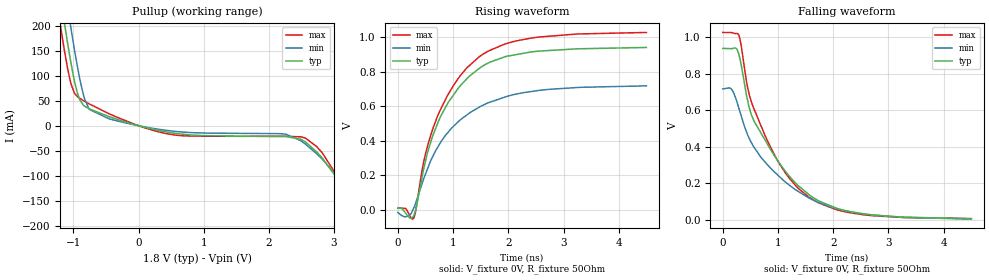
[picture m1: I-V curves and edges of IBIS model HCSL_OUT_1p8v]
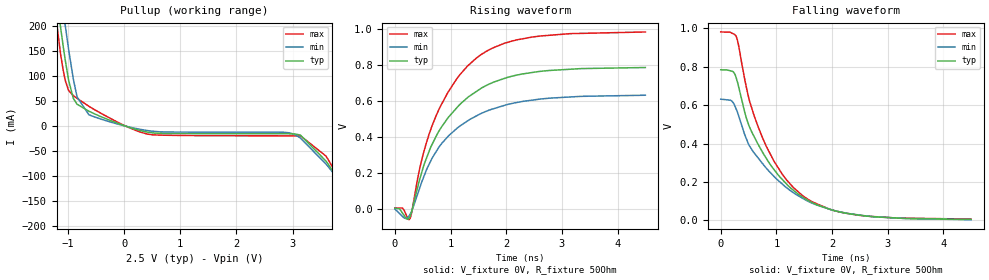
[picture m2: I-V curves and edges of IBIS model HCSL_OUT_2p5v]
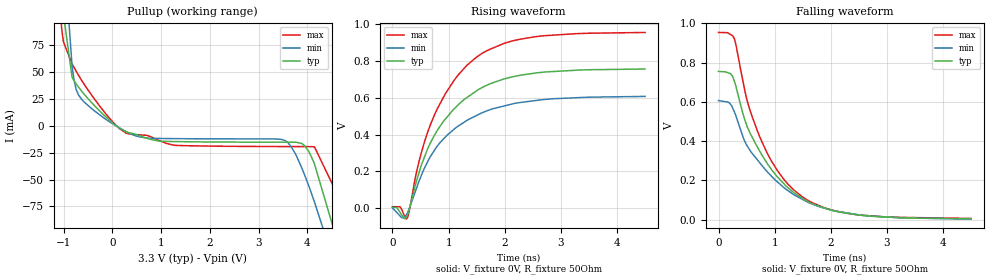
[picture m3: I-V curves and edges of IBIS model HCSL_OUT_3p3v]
|Texas Instruments Incorporated
|Storage Products Group
| Marketing part#   Voltage Range   Package-type   #pins
| CDCUN1208LP   1.7 to  3.63V   QFN   32
[IBIS Ver]   4.0
[File name]   cdcun1208lp.ibs
[File Rev]   1.1
[Date]   04/12/2012
[Source]   Texas Instruments Incorporated.
|   Analog-eLab, HPA
|   12500 TI Blvd
|   Dallas, TX -75243
|   For Support e-mail: elab_ibis@list.ti.com
[Notes]
|-Revision History:
| 1.0: 4/12/2012
| - Initial version of the model
| - Initial Model generated from simulations in TISPICE
| - No syntax warnings or errors based on the
| committee parser checker
| For UNIV_IN2 model, the internal on-chip 50 ohm termination to ground (for
| a HCSL input) and 50 ohm termination to 1.2V (for
| a LVDS input) are not represented in this file. It is recommended
| that a user,who wished to see the benefit of these on-chip terminations,
| implement an appropriate termination explicitly on the final simulation
| level as needed.
[Disclaimer]
 This product is designed as an aid for customers of Texas Instruments.
 No warranties, either expressed or implied, with respect to this third
 party software (if any) or with respect to its fitness for any
 particular purpose is claimed by Texas Instruments or the author. The
 software (if any) is provided solely on an "as is" basis. The entire
 risk as to its quality and performance is with the customer
[Copyright] (C) Copyright 2012 Texas Instruments Incorporated.
   All rights reserved.
|   Component  CDCUN1208LP
[Component]   CDCUN1208LP
[Manufacturer]   Texas Instruments Incorporated
[Package]
| 32-pin QFN
|   typ   min   max
R_pkg   0.44   0.40   0.47
L_pkg   0.734nH   0.634nH   0.824nH
C_pkg   185fF   175fF   195fF
[Pin]   signal_name   model_name   R_pin   L_pin   C_pin
1   DIVIDE   NC   NA   NA   NA
2   INSEL   NC   NA   NA   NA
3   IN1P   UNIV_IN2   NA   NA   NA
4   IN1N   UNIV_IN2   NA   NA   NA
5   VDD   POWER   NA   NA   NA
6   IN2P   UNIV_IN2   NA   NA   NA
7   IN2N   UNIV_IN2   NA   NA   NA
8   ITTP   NC   NA   NA   NA
9   OUT1P   UNIV_OUT   NA   NA   NA
10   OUTIN   UNIV_OUT   NA   NA   NA
11   VDDO1   POWER   NA   NA   NA
12   OUT2P   UNIV_OUT   NA   NA   NA
13   OUT2N   UNIV_OUT   NA   NA   NA
14   VDDO2   POWER   NA   NA   NA
15   OUT3P   UNIV_OUT   NA   NA   NA
16   OUT3N   UNIV_OUT   NA   NA   NA
17   OUT4P   UNIV_OUT   NA   NA   NA
18   OUT4N   UNIV_OUT   NA   NA   NA
19   OTTP   NC   NA   NA   NA
20   OUT5P   UNIV_OUT   NA   NA   NA
21   OUT5N   UNIV_OUT   NA   NA   NA
22   VDDO3   POWER   NA   NA   NA
23   OUT6P   UNIV_OUT   NA   NA   NA
24   OUT6N   UNIV_OUT   NA   NA   NA
25   OUT7P   UNIV_OUT   NA   NA   NA
26   OUT7N   UNIV_OUT   NA   NA   NA
27   VDDO4   POWER   NA   NA   NA
28   OUT8P   UNIV_OUT   NA   NA   NA
29   OUT8N   UNIV_OUT   NA   NA   NA
30   MODE   NC   NA   NA   NA
31   ERC   NC   NA   NA   NA
32   OE   NC   NA   NA   NA
[Diff Pin]  inv_pin  vdiff  tdelay_typ tdelay_min tdelay_max
3   4   200mV   NA   NA   NA
6   7   200mV   NA   NA   NA
9   10   NA   NA   NA   NA
12   13   NA   NA   NA   NA
15   16   NA   NA   NA   NA
17   18   NA   NA   NA   NA
20   21   NA   NA   NA   NA
23   24   NA   NA   NA   NA
25   26   NA   NA   NA   NA
28   29   NA   NA   NA   NA
[Model Selector]   UNIV_OUT
HCSL_OUT_1p8v   HCSL driver w/ 1.8V supply
HCSL_OUT_2p5v   HCSL driver w/ 2.5V supply
HCSL_OUT_3p3v   HCSL driver w/ 3.3V supply
LVCMOS_OUT_1p8v   LVCMOS driver w/ 1.8V supply
LVCMOS_OUT_2p5v   LVCMOS driver w/ 2.5V supply
LVCMOS_OUT_3p3v   LVCMOS driver w/ 3.3V supply
LVDS_OUT_1p8v   LVDS driver w/ 1.8V supply
LVDS_OUT_2p5v   LVDS driver w/ 2.5V supply
LVDS_OUT_3p3v   LVDS driver w/ 3.3V supply
[Model Selector]   IN1
IN1_1p8v   input1 w/ 1.8V supply
IN1_2p5v   input1 w/ 2.5V supply
IN1_3p3v   input1 w/ 3.3V supply
[Model Selector]   UNIV_IN2
UNIVIN2_1p8v   Universal input w/ 1.8V supply
UNIVIN2_2p5v   Universal input w/ 2.5V supply
UNIVIN2_3p3v   Universal input w/ 3.3V supply
| Models and submodels in the file (15): HCSL_OUT_1p8v (Open_source), HCSL_OUT_2p5v (Open_source), HCSL_OUT_3p3v (Open_source), LVCMOS_OUT_1p8v (Output), LVCMOS_OUT_2p5v (Output), LVCMOS_OUT_3p3v (Output), LVDS_OUT_1p8v (Output), LVDS_OUT_2p5v (Output), LVDS_OUT_3p3v (Output), IN1_1p8v (Input), IN1_2p5v (Input), IN1_3p3v (Input), UNIVIN2_1p8v (Input), UNIVIN2_2p5v (Input), UNIVIN2_3p3v (Input)
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[Model]   HCSL_OUT_1p8v
Model_type   Open_source
Polarity   Non-Inverting
Vmeas = 0.35
Vref = 0
Cref = 0pF
Rref = 50
|   typ   min   max
C_comp   1pF   1pF   1pF
[Voltage Range]   1.8   1.7   1.9
[Temperature Range]   27   105   -40
[Pullup Reference]   1.8   1.7   1.9
[Pulldown Reference]   0   0   0
[Power Clamp Reference]   1.8   1.7   1.9
[GND Clamp Reference]   0   0   0
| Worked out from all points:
|   slope of the pullup table from 0 to 0.27 V, typ, clamps not added: 31.8 ohm
|   falling waveform, V_fixture 0V, R_fixture 50Ohm: 20-80 % time 956ps typ, 1.08ns min, 858ps max; typ from 0.939 V to 0.007 V
|   rising waveform, V_fixture 0V, R_fixture 50Ohm: 20-80 % time 792ps typ, 932ps min, 824ps max; typ from 0.008 V to 0.94 V
[Pullup]
|   Voltage   I(typ)   I(min)   I(max)
-1.8V     821.8mA    898.3mA    762.4mA
-1.201V   258.7mA    335mA      200.6mA
-1.147V   211.9mA    287.1mA    156.2mA
-1.049V   133.4mA    203.7mA    89.72mA
-941.4mV  66.24mA    119.5mA    58.45mA
-828mV    38.99mA    53.29mA    48.86mA
-450mV    18.07mA    13.64mA    23.75mA
565.2mV   -15.11mA   -11.22mA   -18.63mA
2.25V     -21.41mA   -16.68mA   -21.21mA
2.563V    -32.41mA   -36.69mA   -24.71mA
2.822V    -64.66mA   -66.78mA   -54.37mA
3.595V    -201.8mA   -185.8mA   -211.9mA
[Ramp]
R_load = 50
|   typ   min   max
dV/dt_r   0.55922/7.89075e-10   0.43998/9.29564e-10   0.610723/8.23426e-10
dV/dt_f   0.559556/9.56565e-10   0.427458/1.07718e-09   0.611668/8.54807e-10
[Falling Waveform]
V_fixture = 0V
V_fixture_min = 0V
V_fixture_max = 0V
R_fixture = 50Ohm
C_fixture = 0F
|   Time   V(typ)   V(min)   V(max)
0s        939.2mV    717.3mV    1.027V
149.3ps   937.9mV    718.6mV    1.026V
286.7ps   911.8mV    617.3mV    1.015V
433.3ps   679.4mV    480.2mV    753.6mV
513.7ps   579.6mV    426.4mV    651.6mV
754.9ps   443.6mV    320.7mV    470.4mV
1.13ns    267.7mV    208.4mV    259.2mV
1.557ns   139.8mV    120.9mV    125.9mV
2.557ns   32.71mV    32.32mV    28.1mV
4.5ns     6.654mV    4.832mV    7.129mV
[Rising Waveform]
V_fixture = 0V
V_fixture_min = 0V
V_fixture_max = 0V
R_fixture = 50Ohm
C_fixture = 0F
|   Time   V(typ)   V(min)   V(max)
0s        7.671mV    -16.04mV   8.717mV
191.1ps   -40.64mV   -37.68mV   -18.56mV
286.7ps   -37.42mV   8.546mV    -50mV
323.5ps   -1.296mV   38.59mV    -7.047mV
488.4ps   263.6mV    195.7mV    305.5mV
709.1ps   490.3mV    354.3mV    533mV
1.081ns   697.6mV    505.3mV    754.2mV
1.476ns   818.8mV    594.2mV    886.2mV
2.401ns   912.9mV    683.7mV    993.3mV
4.5ns     939.7mV    717.3mV    1.027V
[Model]   HCSL_OUT_2p5v
Model_type   Open_source
Polarity   Non-Inverting
Vmeas = 0.35
Vref = 0
Cref = 0pF
Rref = 50
|   typ   min   max
C_comp   1pF   1pF   1pF
[Voltage Range]   2.5   2.375   2.625
[Temperature Range]   27   105   -40
[Pullup Reference]   2.5   2.375   2.625
[Pulldown Reference]   0   0   0
[Power Clamp Reference]   2.5   2.375   2.625
[GND Clamp Reference]   0   0   0
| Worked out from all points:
|   slope of the pullup table from 0 to 0.375 V, typ, clamps not added: 31.2 ohm
|   falling waveform, V_fixture 0V, R_fixture 50Ohm: 20-80 % time 912ps typ, 1.02ns min, 814ps max; typ from 0.785 V to 0.005 V
|   rising waveform, V_fixture 0V, R_fixture 50Ohm: 20-80 % time 911ps typ, 939ps min, 857ps max; typ from 0.006 V to 0.786 V
[Pullup]
|   Voltage   I(typ)   I(min)   I(max)
-2.5V     1.505A     1.579A     1.448A
-1.532V   565.6mA    642.9mA    505.5mA
-1.127V   196.6mA    270.7mA    143.2mA
-1.045V   131.4mA    200.6mA    90.94mA
-902.5mV  55.02mA    94.2mA     60.52mA
-835mV    43.2mA     57.78mA    54.99mA
-625mV    29.29mA    22.18mA    39.09mA
290mV     -9.445mA   -7.035mA   -12.41mA
3.14V     -18.86mA   -24.81mA   -20.12mA
3.59V     -70.25mA   -76.18mA   -60.37mA
4.287V    -195.9mA   -190.4mA   -203.8mA
4.992V    -768mA     -777.7mA   -749.1mA
[Ramp]
R_load = 50
|   typ   min   max
dV/dt_r   0.467952/9.08792e-10   0.378244/9.34994e-10   0.584659/8.56467e-10
dV/dt_f   0.468123/9.123e-10   0.376892/1.01835e-09   0.585226/8.12261e-10
[Falling Waveform]
V_fixture = 0V
V_fixture_min = 0V
V_fixture_max = 0V
R_fixture = 50Ohm
C_fixture = 0F
|   Time   V(typ)   V(min)   V(max)
0s        784.7mV    631.6mV    981.8mV
200.5ps   777.6mV    621.5mV    975.7mV
274.8ps   745.4mV    582.2mV    960.8mV
509.1ps   492.4mV    391.9mV    631.3mV
750.5ps   355.6mV    296.1mV    430.6mV
1.11ns    211.7mV    188mV      238.4mV
1.463ns   123.1mV    116.3mV    130.6mV
1.958ns   57.71mV    57.89mV    57.69mV
2.461ns   28.03mV    28.99mV    27.14mV
4.5ns     4.501mV    3.398mV    6.447mV
[Rising Waveform]
V_fixture = 0V
V_fixture_min = 0V
V_fixture_max = 0V
R_fixture = 50Ohm
C_fixture = 0F
|   Time   V(typ)   V(min)   V(max)
0s        5.615mV    1.546mV    8.04mV
137.7ps   -21.63mV   -39.82mV   6.73mV
210.1ps   -53.53mV   -49.93mV   -35.56mV
267.6ps   -42.09mV   -30.85mV   -53.64mV
491.4ps   213.8mV    158mV      285.1mV
750.5ps   410.1mV    324.2mV    525.7mV
1.11ns    561.7mV    447.3mV    722mV
1.551ns   670.9mV    531.1mV    857.5mV
2.461ns   757.6mV    604.5mV    954mV
4.5ns     785.5mV    632mV      982.5mV
[Model]   HCSL_OUT_3p3v
Model_type   Open_source
Polarity   Non-Inverting
Vmeas = 0.35
Vref = 0
Cref = 0pF
Rref = 50
|   typ   min   max
C_comp   1pF   1pF   1pF
[Voltage Range]   3.3   2.97   3.63
[Temperature Range]   27   105   -40
[Pullup Reference]   3.3   2.97   3.63
[Pulldown Reference]   0   0   0
[Power Clamp Reference]   3.3   2.97   3.63
[GND Clamp Reference]   0   0   0
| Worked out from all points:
|   slope of the pullup table from 0 to 0.495 V, typ, clamps not added: 44.4 ohm
|   falling waveform, V_fixture 0V, R_fixture 50Ohm: 20-80 % time 894ps typ, 1ns min, 798ps max; typ from 0.755 V to 0.004 V
|   rising waveform, V_fixture 0V, R_fixture 50Ohm: 20-80 % time 914ps typ, 937ps min, 864ps max; typ from 0.005 V to 0.756 V
[Pullup]
|   Voltage   I(typ)   I(min)   I(max)
-3.3V     2.293A     2.365A     2.238A
-1.043V   130.8mA    199.3mA    92.26mA
-1.003V   103.8mA    167.4mA    78.11mA
-825mV    44.96mA    55.2mA     57.46mA
-686.4mV  35.51mA    28.08mA    46.44mA
283.8mV   -5.615mA   -5.555mA   -6.779mA
3.541V    -15.29mA   -13.74mA   -19.34mA
3.937V    -18.15mA   -44.83mA   -19.39mA
4.145V    -35.25mA   -70.54mA   -19.52mA
4.62V     -108.1mA   -137.4mA   -64.22mA
4.808V    -141.4mA   -168.2mA   -100.1mA
6.59V     -1.543A    -1.748A    -1.326A
[Ramp]
R_load = 50
|   typ   min   max
dV/dt_r   0.450607/9.05593e-10   0.363664/9.3445e-10   0.568417/8.6254e-10
dV/dt_f   0.450715/8.95406e-10   0.362311/1.00092e-09   0.568823/7.98193e-10
[Falling Waveform]
V_fixture = 0V
V_fixture_min = 0V
V_fixture_max = 0V
R_fixture = 50Ohm
C_fixture = 0F
|   Time   V(typ)   V(min)   V(max)
0s        755.4mV    607mV      954.2mV
197.9ps   745.6mV    594.1mV    946.6mV
275.8ps   710.9mV    554mV      926.6mV
527.8ps   462.7mV    368.4mV    588.5mV
862.3ps   289.2mV    246.2mV    342.2mV
1.171ns   181.3mV    162.1mV    202.8mV
1.493ns   109.5mV    103.7mV    116.5mV
1.886ns   59.76mV    58.78mV    60.62mV
2.387ns   28.5mV     29.66mV    28.25mV
4.5ns     4.232mV    3.101mV    6.161mV
[Rising Waveform]
V_fixture = 0V
V_fixture_min = 0V
V_fixture_max = 0V
R_fixture = 50Ohm
C_fixture = 0F
|   Time   V(typ)   V(min)   V(max)
0s        5.333mV    1.237mV    7.669mV
160.2ps   -35.28mV   -50.73mV   -4.912mV
263.7ps   -40.27mV   -27.44mV   -54.11mV
491.6ps   211.2mV    160.5mV    276.2mV
739.8ps   391.9mV    310.8mV    501.3mV
1.104ns   541.7mV    430.8mV    697.4mV
1.493ns   636.5mV    503.2mV    819.9mV
2ns       703.4mV    556.2mV    897.2mV
2.535ns   733.9mV    584.4mV    931.4mV
4.5ns     756.3mV    607.3mV    955mV
